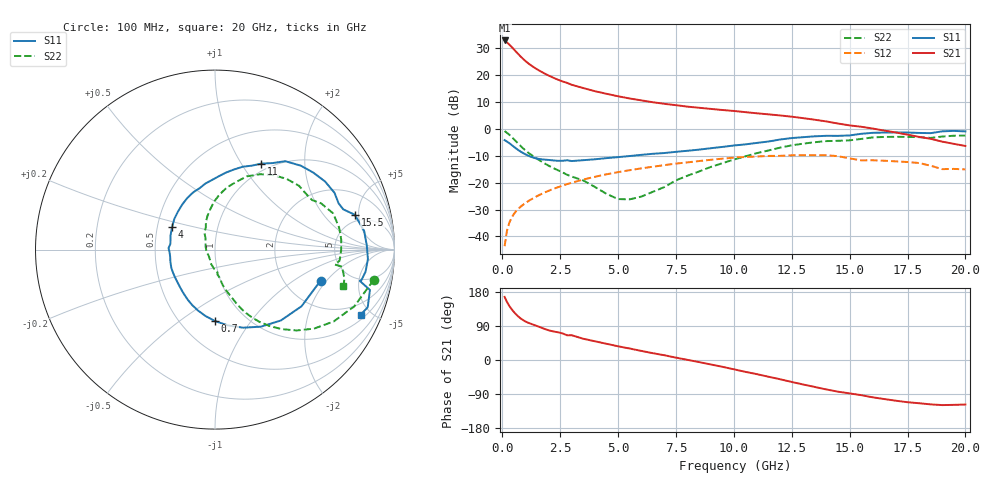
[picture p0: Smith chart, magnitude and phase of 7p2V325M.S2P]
! Infineon Technologies  Discrete & RF Semiconductors
! bfp620
! VCE =  2.3 V,  IC =  25 mA
! Common Emitter S-Parameters:  Sep 2002
# GHz  S  MA  R  50
!  f  S11  S21  S12  S22
! GHz  MAG  ANG  MAG  ANG  MAG  ANG  MAG  ANG
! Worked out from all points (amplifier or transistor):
!   59 points, 100 MHz to 20 GHz, reference 50 ohm
!   highest |S21| = 32.7 dB at 100 MHz (marker M1)
!   |S21| within 3 dB of that: start of sweep to 468.6 MHz
!   unconditionally stable (mu >= 1): 2.934 GHz to 9.92 GHz; 17.18 GHz to end of sweep
!   at 1 GHz: K = 0.75, MSG = 26.4 dB, |S12| = -27.6 dB
!   at 5.5 GHz: K = 1.04, MAG = 12.1 dB, |S12| = -15.4 dB
!   at 20 GHz: K = 1.26, MAG = 1.3 dB, |S12| = -15.1 dB
!   S11 on the Smith chart (normalised r, x): 100 MHz: 3.13, -1.73; 700 MHz: 0.73, -0.69; 4 GHz: 0.60, +0.16; 11 GHz: 0.90, +1.23; 15.5 GHz: 4.11, +4.49; 20 GHz: 1.26, -4.36
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0.1  0.613 -16.4  43.33 166.5  0.0066 51.9  0.9003 -10.8
0.2  0.5764 -33.2  39.8 153.5  0.0126 63.4  0.8378 -22.2
0.3  0.5391 -47.1  36.38 143.0  0.0178 64.2  0.773 -31.2
0.4  0.5 -59.2  32.97 134.3  0.0222 63.1  0.7058 -38.6
0.5  0.4621 -70.3  29.68 126.7  0.0261 61.6  0.6396 -44.8
0.6  0.4279 -80.5  26.65 120.1  0.0296 60.4  0.5775 -50.1
0.7  0.3984 -89.9  23.97 114.3  0.0328 59.4  0.5217 -54.6
0.8  0.3734 -98.3  21.65 109.4  0.0359 58.7  0.4728 -58.4
1  0.334 -112.4  18.01 101.7  0.0417 57.9  0.395 -63.8
1.2  0.3051 -123.6  15.39 96.4  0.0474 57.3  0.3383 -67.3
1.6  0.2735 -142.4  11.94 87.4  0.0588 56.0  0.2602 -72.5
2  0.2628 -158.3  9.687 78.4  0.0703 54.0  0.2059 -77.4
2.4  0.253 -170.9  8.112 73.2  0.0818 51.8  0.1696 -79.6
3.5  0.2601 162.1  5.66 56.0  0.1139 43.5  0.1092 -91.9
4  0.2701 152.4  4.959 49.4  0.128 39.3  0.0829 -105.1
7  0.3531 103.9  2.889 12.5  0.2105 12.3  0.0825 129.9
10.5  0.5112 66.2  2.025 -31.3  0.2983 -26.2  0.3068 85.4
11  0.5444 61.7  1.927 -37.4  0.3046 -31.5  0.3518 79.3
13.5  0.7213 31.7  1.464 -71.2  0.3215 -62.0  0.5606 44.7
15.5  0.8028 14.0  1.085 -92.8  0.258 -84.0  0.6446 23.6
17  0.8536 -3.5  0.85 -107.5  0.2473 -93.9  0.7055 4.5
20  0.8894 -24.0  0.477 -117.5  0.1755 -103.6  0.7433 -15.7
